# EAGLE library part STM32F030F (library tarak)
STM32F050F4P6
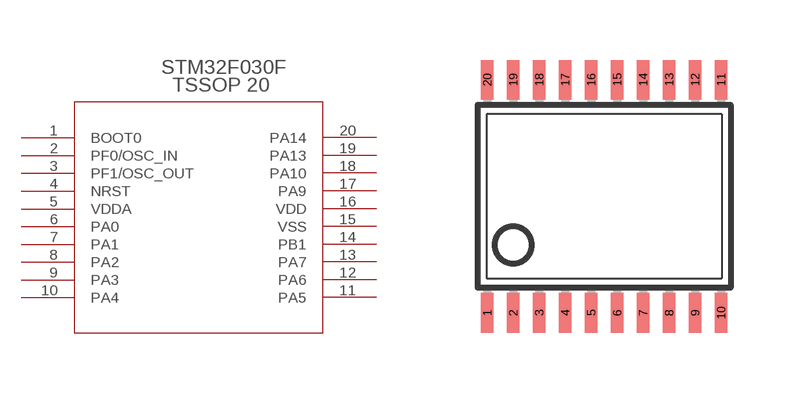
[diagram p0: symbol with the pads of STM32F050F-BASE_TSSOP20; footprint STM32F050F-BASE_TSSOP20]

Designator prefix -

## STM32F030F  [STM32F050F-BASE_TSSOP20]
1  BOOT0  pas
2  PF0/OSC_IN  pas
3  PF1/OSC_OUT  pas
4  NRST  pas
5  VDDA  pas
6  PA0  pas
7  PA1  pas
8  PA2  pas
9  PA3  pas
10  PA4  pas
11  PA5  pas
12  PA6  pas
13  PA7  pas
14  PB1  pas
15  VSS  pas
16  VDD  pas
17  PA9  pas
18  PA10  pas
19  PA13  pas
20  PA14  pas

## Footprint STM32F050F-BASE_TSSOP20 (pad centres in mm)
Thin Shrink Small Outline Plastic 20
smd 0.305 x 0.991: 1 -2.925,-2.918; 2 -2.275,-2.918; 3 -1.625,-2.918; 4 -0.975,-2.918; 5 -0.325,-2.918; 6 0.325,-2.918; 7 0.975,-2.918; 8 1.625,-2.918; 9 2.275,-2.918; 10 2.925,-2.918; 11 2.925,2.918; 12 2.275,2.918; 13 1.625,2.918; 14 0.975,2.918; 15 0.325,2.918; 16 -0.325,2.918; 17 -0.975,2.918; 18 -1.625,2.918; 19 -2.275,2.918; 20 -2.925,2.918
